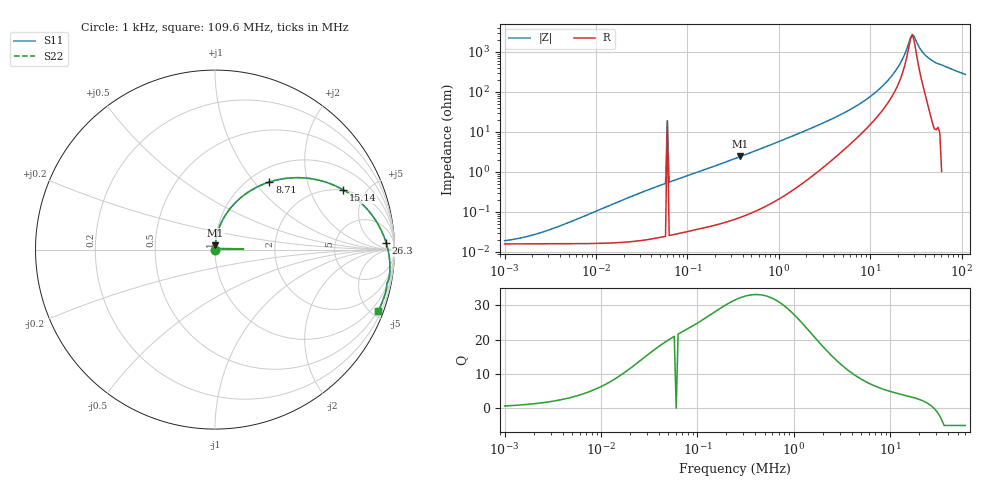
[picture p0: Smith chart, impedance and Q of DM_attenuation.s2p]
! EM Consulting and Software
! Touchstone file was created on 2026-03-05  19:00:36
# HZ S RI R 50.0000
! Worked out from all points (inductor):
!   253 points, 1 kHz to 109.6 MHz, reference 50 ohm
!   read as one part in series: L = 1.65 uH near 4.786 kHz
!   highest Q = 33.1 at 380.2 kHz (marker M1), where L = 1.02 uH
!   self-resonance near 27.54 MHz
!   S11 on the Smith chart (normalised r, x): 1 kHz: 1.00, +0.00; 8.71 MHz: 1.22, +1.20; 15.14 MHz: 1.97, +3.47; 26.3 MHz: 26, +21; 109.6 MHz: 0.43, -5.44
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1000  0.000159 0.000106  0.9998 -0.000106  0.9998 -0.000106  0.000159 0.000106
2290.868  0.00016 0.000239  0.9998 -0.000239  0.9998 -0.000239  0.00016 0.000239
6918.31  0.000162 0.000717  0.9998 -0.000717  0.9998 -0.000717  0.000162 0.000717
47863.01  0.000247 0.00443  0.9998 -0.00443  0.9998 -0.00443  0.000247 0.00443
57543.99  0.000273 0.00516  0.9997 -0.00516  0.9997 -0.00516  0.000273 0.00516
60255.96  0.159 0.0043  0.841 -0.0043  0.841 -0.0043  0.159 0.0043
63095.73  0.000288 0.00556  0.9997 -0.00556  0.9997 -0.00556  0.000288 0.00556
331131.1  0.00112 0.0215  0.9989 -0.0215  0.9989 -0.0215  0.00112 0.0215
380189.4  0.00132 0.0243  0.9987 -0.0243  0.9987 -0.0243  0.00132 0.0243
2290868  0.0228 0.1216  0.9772 -0.1216  0.9772 -0.1216  0.0228 0.1216
5011872  0.1019 0.2492  0.8981 -0.2492  0.8981 -0.2492  0.1019 0.2492
8709636  0.3029 0.3766  0.6971 -0.3766  0.6971 -0.3766  0.3029 0.3766
1.148154e7  0.4943 0.3998  0.5057 -0.3998  0.5057 -0.3998  0.4943 0.3998
1.513561e7  0.7149 0.333  0.2851 -0.333  0.2851 -0.333  0.7149 0.333
1.659587e7  0.7797 0.2895  0.2203 -0.2895  0.2203 -0.2895  0.7797 0.2895
2.187762e7  0.9133 0.1324  0.0867 -0.1324  0.0867 -0.1324  0.9133 0.1324
2.630268e7  0.9543 0.0356  0.0457 -0.0356  0.0457 -0.0356  0.9543 0.0356
2.884032e7  0.9649 -0.00565  0.0351 0.00565  0.0351 0.00565  0.9649 -0.00565
3.630781e7  0.9747 -0.0883  0.0253 0.0883  0.0253 0.0883  0.9747 -0.0883
4.365158e7  0.9724 -0.1388  0.0276 0.1388  0.0276 0.1388  0.9724 -0.1388
5.248075e7  0.9619 -0.1811  0.0381 0.1811  0.0381 0.1811  0.9619 -0.1811
1.096478e8  0.9098 -0.344  0.0902 0.344  0.0902 0.344  0.9098 -0.344
